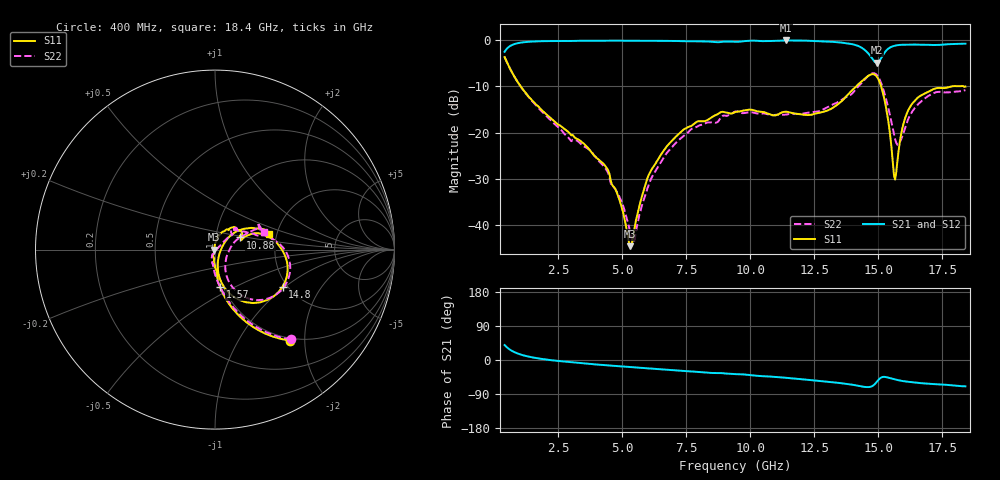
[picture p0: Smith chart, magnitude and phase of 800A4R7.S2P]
!  American Technical Ceramics  Date:  12/17/08
!  One Norden Lane
!  Huntington Station,  NY.  11746-2102
!  Tel:  (631) 622-4700  Fax:  (631) 622-4748
!  Part Number  800A4R7
!  Description: Broardband capacitor  Mounting Orientation: Vertical
!  Application:
# GHZ S DB R 50
! Freq  |S11|  S11 Ph  |S21|  S21 Ph  |S12|  S12 Ph  |S22|  S22 Ph
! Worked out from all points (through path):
!   401 points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, 400 MHz to 18.4 GHz, reference 50 ohm
!   highest |S21| = -0.06 dB at 11.38 GHz (marker M1); lowest = -4.9 dB at 14.94 GHz (marker M2)
!   group delay of S21, straight-line fit = 12.8 ps
!   lowest |S11| = -44.5 dB at 5.305 GHz (marker M3), VSWR 1.01, Z = 49.4 - j0.106 ohm
!   |S11| at or under -10 dB: 1.031 GHz to 14.13 GHz (13.1 GHz wide, 173 % of centre); 15.11 GHz to 17.85 GHz (2.746 GHz wide, 16.7 % of centre); 18.335 GHz to end of sweep
!   |S22| runs from -43.7 to -3.7 dB; largest |S21 - S12| = 0.0026
!   S11 on the Smith chart (normalised r, x): 400 MHz: 0.95, -1.70; 1.57 GHz: 0.97, -0.42; 10.88 GHz: 1.31, +0.18; 14.8 GHz: 1.90, -0.96; 18.4 GHz: 1.83, +0.35
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0.4  -3.66 -50.7  -2.51 39.4  -2.50 39.4  -3.66 -49.7
0.85  -8.49 -71.1  -0.73 18.7  -0.72 18.7  -8.51 -69.7
1.57  -13.60 -82.2  -0.28 5.9  -0.27 5.8  -13.70 -82.7
3.415  -22.00 -92.0  -0.12 -8.6  -0.12 -8.6  -22.56 -102.1
4.405  -27.72 -102.8  -0.13 -14.1  -0.12 -14.1  -28.25 -115.7
5.305  -44.49 -169.6  -0.13 -18.6  -0.12 -18.7  -41.45 -69.2
5.485  -40.33 119.9  -0.13 -19.4  -0.13 -19.5  -42.98 -11.1
5.935  -30.49 91.7  -0.11 -21.6  -0.11 -21.7  -32.86 33.3
6.43  -25.41 81.0  -0.14 -24.2  -0.14 -24.2  -27.06 40.2
7.465  -19.06 65.1  -0.23 -29.2  -0.23 -29.3  -20.38 42.6
9.4  -15.56 41.7  -0.35 -37.2  -0.36 -37.4  -15.44 46.0
10.885  -16.23 26.1  -0.16 -44.2  -0.17 -44.2  -16.18 46.1
11.38  -15.45 24.6  -0.06 -47.0  -0.07 -47.0  -16.07 46.1
12.415  -16.06 21.7  -0.15 -53.4  -0.15 -53.4  -15.55 38.0
14.08  -10.29 13.4  -1.01 -66.5  -1.01 -66.4  -10.87 16.1
14.8  -7.34 -28.6  -4.28 -67.2  -4.29 -67.2  -7.13 -22.8
14.935  -7.85 -43.8  -4.87 -57.9  -4.87 -57.8  -7.49 -36.8
15.43  -19.15 -81.5  -1.67 -47.4  -1.67 -47.4  -15.61 -66.4
15.655  -30.11 -14.1  -1.17 -51.5  -1.18 -51.5  -21.38 -45.2
16.015  -17.39 41.5  -0.99 -56.2  -0.99 -56.2  -19.40 18.4
16.375  -13.38 33.5  -0.96 -59.1  -0.97 -59.0  -15.00 26.4
18.4  -10.02 15.9  -0.76 -69.5  -0.77 -69.5  -10.79 19.6
